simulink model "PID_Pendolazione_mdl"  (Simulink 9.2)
settings: Solver=ode45  StartTime=0.0  StopTime=10.0  RelTol=1e-3  EnableMultiTasking=on
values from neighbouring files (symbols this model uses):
  Den = DEN{1}    [PID_Pendolazione.m]
  K = M0*(4/3+R/4)/(N*t0)    [Choen_Coon.m]    (also in PID_PARAMETRI.m = C0/M0; PID_Tuning_Example.m = 0.6*K0; Ziegler.m = 0.6*K0)
  Num = NUM{1}    [PID_Pendolazione.m]
  r0 = 1    [PID_Pendolazione.m]
  U_max = 10    [PID_Pendolazione.m]

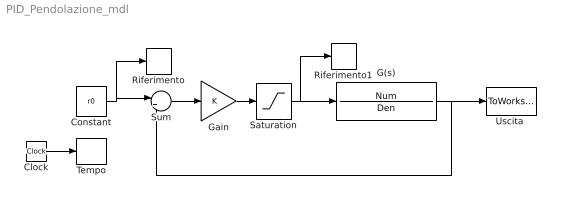
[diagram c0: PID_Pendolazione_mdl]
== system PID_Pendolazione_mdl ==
  Clock : Clock
  Constant : Constant  Value=r0
  G(s) : TransferFcn  Numerator=Num  Denominator=Den
  Gain : Gain  Gain=K
  Riferimento : ToWorkspace  VariableName=rt  SampleTime=-1
  Riferimento1 : ToWorkspace  VariableName=ut  SampleTime=-1
  Saturation : Saturate  UpperLimit=U_max  LowerLimit=-U_max
  Sum : Sum  Inputs=|+-
  Tempo : ToWorkspace  VariableName=t  SampleTime=-1
  "Uscita " : ToWorkspace  VariableName=yt  SampleTime=-1
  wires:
  Constant/1 -> Sum/1, Riferimento/1
  Clock/1 -> Tempo/1
  Gain/1 -> Saturation/1
  Sum/1 -> Gain/1
  G(s)/1 -> "Uscita "/1, Sum/2
  Saturation/1 -> Riferimento1/1, G(s)/1
